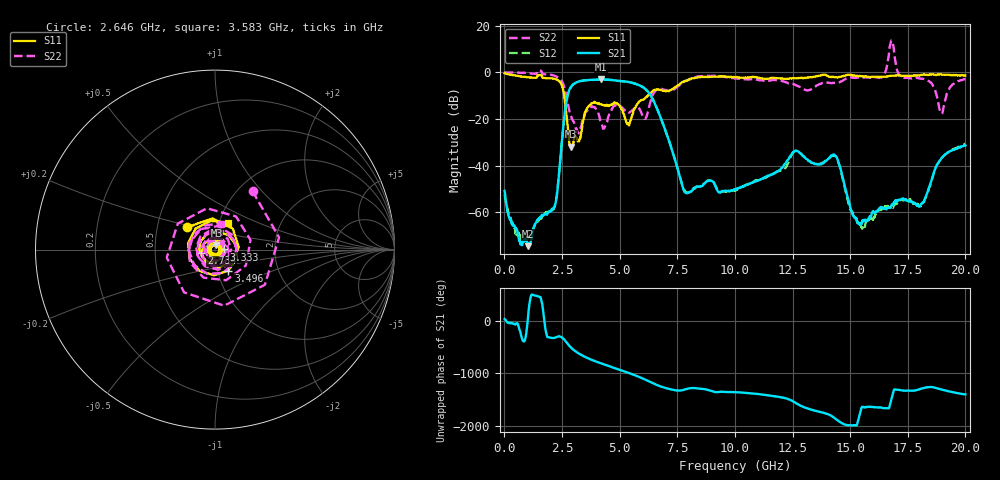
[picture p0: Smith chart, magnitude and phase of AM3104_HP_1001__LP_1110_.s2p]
!Created with skrf (http://scikit-rf.org).
# Hz S RI R 50.0
!freq ReS11 ImS11 ReS21 ImS21 ReS12 ImS12 ReS22 ImS22
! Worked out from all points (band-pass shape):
!   1601 points, 10 MHz to 20 GHz, reference 50 ohm
!   highest |S21| = -3.05 dB at 4.195 GHz (marker M1); lowest = -74.4 dB at 1.01 GHz (marker M2)
!   |S21| within 3 dB of the highest: 2.907 GHz to 5.956 GHz (3.049 GHz wide, 68.8 % of centre)
!   lowest |S11| = -31.8 dB at 2.871 GHz (marker M3), VSWR 1.05, Z = 50.7 + j2.48 ohm
!   |S11| at or under -10 dB: 2.597 GHz to 6.223 GHz (3.625 GHz wide, 82.2 % of centre)
!   |S22| runs from -26.1 to 13.6 dB; largest |S21 - S12| = 0.077
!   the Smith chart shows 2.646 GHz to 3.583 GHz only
!   S11 on the Smith chart (normalised r, x): 2.646 GHz: 0.71, +0.19; 2.734 GHz: 0.86, -0.04; 3.333 GHz: 1.11, +0.00; 3.496 GHz: 1.13, -0.27; 3.583 GHz: 1.10, +0.34
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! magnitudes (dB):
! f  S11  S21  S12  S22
! 10 MHz  -0.4  -50.8  -52.1  -0.1
! 1.01 GHz  -2.2  -74.4  -70.6  -0.4
! 2.171 GHz  -2.8  -57.6  -57.6  -1.5
! 2.646 GHz  -14.1  -15.5  -15.5  -8.3
! 2.734 GHz  -22.1  -10.3  -10.3  -12.6
! 2.871 GHz  -31.8  -6.5  -6.6  -18.3
! 3.333 GHz  -26.0  -3.7  -3.7  -23.1
! 3.346 GHz  -25.3  -3.6  -3.7  -22.7
! 3.496 GHz  -17.2  -3.4  -3.5  -17.7
! 3.583 GHz  -15.6  -3.3  -3.4  -16.6
! 4.195 GHz  -13.8  -3.0  -3.1  -21.6
! 5.382 GHz  -22.5  -4.2  -4.2  -17.1
! 6.682 GHz  -7.3  -17.0  -17.0  -7.1
! 7.856 GHz  -3.7  -51.6  -51.2  -3.8
! 10.01 GHz  -2.2  -50.3  -50.7  -2.7
! 13.34 GHz  -2.2  -38.7  -38.8  -7.1
! 14.38 GHz  -2.1  -35.9  -36.2  -4.5
! 15.54 GHz  -1.6  -63.3  -66.3  -2.2
! 16.68 GHz  -1.6  -57.9  -57.8  7.3
! 18.09 GHz  -1.0  -56.3  -57.0  -2.7
! 18.95 GHz  -0.9  -36.9  -37.0  -17.5
! 20 GHz  -1.3  -31.3  -30.6  -2.9
